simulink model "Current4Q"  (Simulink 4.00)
settings: Solver=ode45  StartTime=0.0  StopTime=0.1  MaxStep=0.000005  RelTol=1e-3
undefined symbols (not defined in the file or in its folder): di, La, Ra, Symmetric, Ts, Ttc, Udc
libraries: simulink3 x1

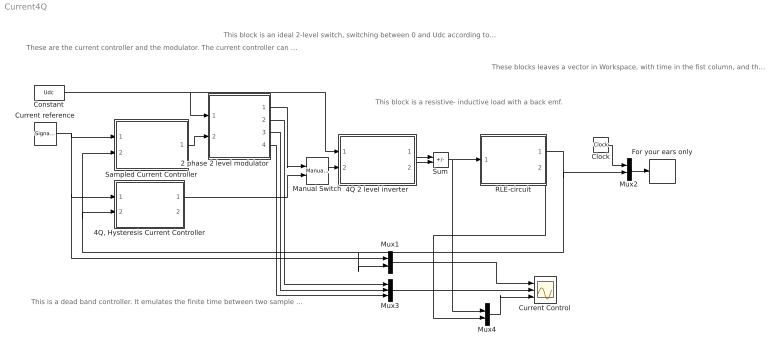
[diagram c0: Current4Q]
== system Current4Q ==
  note: These are the current controller and the modulator. The current controller can emulate several types of controllers.The most didactic is the "fast" but the most realistic is the "slow" and the "slow with Smith Predictor".
  note: This is a dead band controller. It emulates the finite time between two sample time instants, and a dead band.
  note: This block is an ideal 2-level switch, switching between 0 and Udc according to the input signal .
  note: This block is a resistive- inductive load with a back emf.
  note: These blocks leaves a vector in Workspace, with time in the fist column, and the current in the second. Use th file "Playsound" to listen to the sound of the converter, IF you have a sound card in your computer. Type: >>playsound(snd(:,1),snd(:,2))
  2 phase 2 level modulator : Subsystem  mask{Ts=Ts, Random=Fixed frequency, Minswitch=Symmetric}
      mask prompts: Ts "Sampling Interval [s]"; Random "Fixed or random frequency"; Minswitch "Symmetric of Minswitch Modulation"
      mask help: Carrier Wave modulator that uses either fixed frequency modulation or random modulation. The fixed frequency modulation uses 1/(2Ts) as modulation frequency. The random modulation selects the modulatio frequency by random every sampling instant. The selection uses either 1/Ts, 1/(2Ts) or 1/(3Ts) as carrier wave frequency.
      mask init:
      | seed=rand
  4Q 2 level inverter : Subsystem
  "4Q, Hysteresis Current Controller" : Subsystem
  Clock : Clock
  Constant : Constant  Value=Udc
  Current reference : SignalGenerator  WaveForm=square  Amplitude=10  Frequency=20  Units=Hertz
  Current Control : Scope  NumInputPorts=3
  For your ears only : ToWorkspace  VariableName=snd  SampleTime=-1  SaveFormat=Array
  Manual Switch : simulink3/Nonlinear/Manual Switch  sw=1  action=0
  Mux1 : Mux  Inputs=2
  Mux2 : Mux  Inputs=2
  Mux3 : Mux  Inputs=3
  Mux4 : Mux  Inputs=2
  RLE-circuit : Subsystem  mask(RLE-circuit){L=La, R=Ra, e0=40, i0=0}
      mask prompts: L "L [H]"; R "R [ohm]"; e0 "Back emf"; i0 "Starting Current"
      mask help: Parametrar
  Sampled Current Controller : Subsystem  mask{R=Ra, L=La, Kp=(La/Ttc+Ra/2), Ti=La/Ra+Ttc/2, Ttc=Ttc, Umax=Udc, Umin=-Udc, e0=40, SlowFast=Slow Computer with Smith Predictor}
      mask prompts: R "Load resistance"; L "Load inductance"; Kp "Controller gain"; Ti "Integral Time Constant"; Ttc "Sampling time [s]"; Umax "Max output signal"; Umin "Min output signal"; e0 "Starting emf"; SlowFast "Controller type"
  Sum : Sum  Inputs=+-  SaturateOnIntegerOverflow=on
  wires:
  RLE-circuit/1(i) -> Mux2/2, "4Q, Hysteresis Current Controller"/2(i), Sampled Current Controller/2(Act), Mux1/2
  Constant/1 -> 4Q 2 level inverter/1(Udc), 2 phase 2 level modulator/1(udc)
  Clock/1 -> Mux2/1
  Mux2/1 -> For your ears only/1
  Mux1/1 -> Current Control/1
  Mux3/1 -> Current Control/2
  Current reference/1 -> Sampled Current Controller/1(Ref), Mux1/1, "4Q, Hysteresis Current Controller"/1(i*)
  4Q 2 level inverter/1(va) -> Sum/1
  4Q 2 level inverter/2(vb) -> Sum/2
  Sum/1 -> Mux4/1, RLE-circuit/1(u)
  2 phase 2 level modulator/1(sa,b) -> Manual Switch/1
  "4Q, Hysteresis Current Controller"/1(sa,b) -> Manual Switch/2
  Manual Switch/1 -> 4Q 2 level inverter/2(sa,b)
  2 phase 2 level modulator/2(va*) -> Mux3/1
  2 phase 2 level modulator/3(vb*) -> Mux3/2
  2 phase 2 level modulator/4(um) -> Mux3/3
  Sampled Current Controller/1(u*) -> 2 phase 2 level modulator/2(u*)
  Mux4/1 -> Current Control/3
  RLE-circuit/2(" e") -> Mux4/2

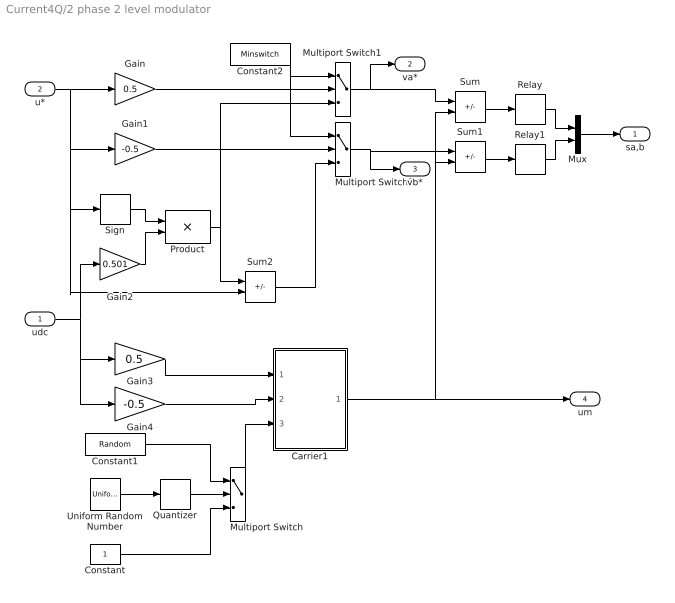
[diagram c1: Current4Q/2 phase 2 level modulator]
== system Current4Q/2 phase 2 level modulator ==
  udc : Inport  Port=1  LatchInput=off
  u* : Inport  Port=2  LatchInput=off
  Carrier1 : Subsystem
  Constant : Constant  Value=1
  Constant1 : Constant  Value=Random
  Constant2 : Constant  Value=Minswitch
  Gain : Gain  Gain=0.5  Multiplication=Element-wise(K.*u)  SaturateOnIntegerOverflow=on
  Gain1 : Gain  Gain=-0.5  Multiplication=Element-wise(K.*u)  SaturateOnIntegerOverflow=on
  Gain2 : Gain  Gain=0.501  Multiplication=Element-wise(K.*u)  SaturateOnIntegerOverflow=on
  Gain3 : Gain  Gain=0.5  Multiplication=Element-wise(K.*u)  SaturateOnIntegerOverflow=on
  Gain4 : Gain  Gain=-0.5  Multiplication=Element-wise(K.*u)  SaturateOnIntegerOverflow=on
  Multiport Switch : MultiPortSwitch  Inputs=2
  Multiport Switch1 : MultiPortSwitch  Inputs=2
  Multiport Switch2 : MultiPortSwitch  Inputs=2
  Mux : Mux  Inputs=2
  Product : Product  Inputs=2  Multiplication=Element-wise(.*)  SaturateOnIntegerOverflow=on
  Quantizer : Quantizer  QuantizationInterval=1  LinearizeAsGain=on
  Relay : Relay  OnSwitchValue=eps  OffSwitchValue=eps  OnOutputValue=1  OffOutputValue=-1
  Relay1 : Relay  OnSwitchValue=eps  OffSwitchValue=eps  OnOutputValue=1  OffOutputValue=-1
  Sign : Signum
  Sum : Sum  Inputs=+-  SaturateOnIntegerOverflow=on
  Sum1 : Sum  Inputs=+-  SaturateOnIntegerOverflow=on
  Sum2 : Sum  Inputs=+-  SaturateOnIntegerOverflow=on
  Uniform Random Number : UniformRandomNumber  Minimum=1  Maximum=3  Seed=seed  SampleTime=Ts
  sa,b : Outport  Port=1  InitialOutput=0
  va* : Outport  Port=2  InitialOutput=0
  vb* : Outport  Port=3  InitialOutput=0
  um : Outport  Port=4  InitialOutput=0
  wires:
  Sum/1 -> Relay/1
  Sum1/1 -> Relay1/1
  u*/1 -> Gain/1, Gain1/1, Sign/1, Sum2/2
  Sign/1 -> Product/1
  udc/1 -> Gain2/1, Gain3/1, Gain4/1
  Gain2/1 -> Product/2
  Product/1 -> Sum2/1, Multiport Switch1/3
  Gain/1 -> Multiport Switch1/2
  Gain1/1 -> Multiport Switch2/2
  Multiport Switch1/1 -> Sum/1, va*/1
  Multiport Switch2/1 -> Sum1/1, vb*/1
  Sum2/1 -> Multiport Switch2/3
  Gain4/1 -> Carrier1/2(Umin)
  Gain3/1 -> Carrier1/1(Umax)
  Quantizer/1 -> Multiport Switch/2
  Uniform Random Number/1 -> Quantizer/1
  Constant/1 -> Multiport Switch/3
  Multiport Switch/1 -> Carrier1/3(x)
  Constant1/1 -> Multiport Switch/1
  Carrier1/1(um) -> Sum1/2, Sum/2, um/1
  Constant2/1 -> Multiport Switch1/1, Multiport Switch2/1
  Relay/1 -> Mux/1
  Relay1/1 -> Mux/2
  Mux/1 -> sa,b/1

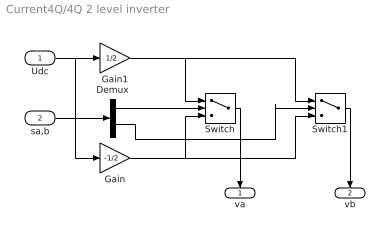
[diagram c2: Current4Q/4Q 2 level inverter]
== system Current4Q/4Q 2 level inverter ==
  Udc : Inport  Port=1  LatchInput=off
  sa,b : Inport  Port=2  LatchInput=off
  Demux : Demux  Outputs=2  BusSelectionMode=off
  Gain : Gain  Gain=-1/2  Multiplication=Element-wise(K.*u)  SaturateOnIntegerOverflow=on
  Gain1 : Gain  Gain=1/2  Multiplication=Element-wise(K.*u)  SaturateOnIntegerOverflow=on
  Switch : Switch  Threshold=0
  Switch1 : Switch  Threshold=0
  va : Outport  Orientation=down  Port=1  InitialOutput=0
  vb : Outport  Orientation=down  Port=2  InitialOutput=0
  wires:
  Gain1/1 -> Switch/1, Switch1/1
  Gain/1 -> Switch/3, Switch1/3
  Switch/1 -> va/1
  Switch1/1 -> vb/1
  Udc/1 -> Gain1/1, Gain/1
  sa,b/1 -> Demux/1
  Demux/1 -> Switch/2
  Demux/2 -> Switch1/2

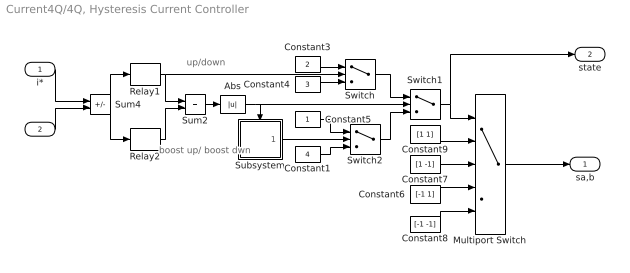
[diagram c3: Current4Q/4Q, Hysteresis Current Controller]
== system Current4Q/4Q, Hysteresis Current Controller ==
  note: up/down
  note: boost up/ boost dwn
  i* : Inport  Port=1  LatchInput=off
  i : Inport  Port=2  LatchInput=off
  Abs : Abs  SaturateOnIntegerOverflow=on
  Constant1 : Constant  Value=4
  Constant3 : Constant  Value=2
  Constant4 : Constant  Value=3
  Constant5 : Constant  Value=1
  Constant6 : Constant  Value=[-1 1]
  Constant7 : Constant  Value=[1 -1]
  Constant8 : Constant  Value=[-1 -1]
  Constant9 : Constant  Value=[1 1]
  Multiport Switch : MultiPortSwitch  Inputs=4
  Relay1 : Relay  OnSwitchValue=di/2  OffSwitchValue=-di/2  OnOutputValue=1  OffOutputValue=-1
  Relay2 : Relay  OnSwitchValue=1.3*di/2  OffSwitchValue=-1.3*di/2  OnOutputValue=1  OffOutputValue=-1
  Subsystem : Subsystem  TreatAsAtomicUnit=on
  Sum2 : Sum  Inputs=++  SaturateOnIntegerOverflow=on
  Sum4 : Sum  Inputs=+-  SaturateOnIntegerOverflow=on
  Switch : Switch  Threshold=0
  Switch1 : Switch  Threshold=1
  Switch2 : Switch  Threshold=0.5
  sa,b : Outport  Port=1
  state : Outport  Port=2
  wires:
  Sum4/1 -> Relay1/1, Relay2/1
  Relay1/1 -> Sum2/1, Switch/2
  Relay2/1 -> Sum2/2
  Sum2/1 -> Abs/1
  Switch/1 -> Switch1/1
  Constant3/1 -> Switch/1
  Constant4/1 -> Switch/3
  Switch1/1 -> Multiport Switch/1, state/1
  Multiport Switch/1 -> sa,b/1
  Abs/1 -> Switch1/2, Subsystem/Trigger
  i*/1 -> Sum4/1
  i/1 -> Sum4/2
  Constant5/1 -> Switch2/1
  Constant1/1 -> Switch2/3
  Switch2/1 -> Switch1/3
  Subsystem/1(Toggle) -> Switch2/2
  Constant6/1 -> Multiport Switch/4
  Constant7/1 -> Multiport Switch/3
  Constant8/1 -> Multiport Switch/5
  Constant9/1 -> Multiport Switch/2

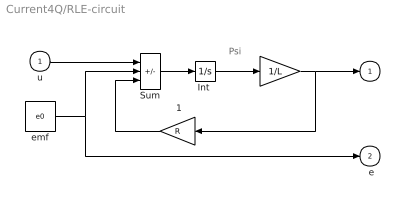
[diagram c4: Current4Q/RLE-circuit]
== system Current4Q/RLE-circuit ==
  note: i
  note: Psi
  u : Inport  Port=1  LatchInput=off
  " " : Gain  Gain=1/L  Multiplication=Element-wise(K.*u)  SaturateOnIntegerOverflow=on
  " 1" : Gain  Orientation=left  Gain=R  Multiplication=Element-wise(K.*u)  SaturateOnIntegerOverflow=on
  "Int " : Integrator  ExternalReset=none  InitialConditionSource=internal  InitialCondition=i0*L  LimitOutput=off  UpperSaturationLimit=inf  LowerSaturationLimit=-inf  ShowSaturationPort=off  ShowStatePort=off  AbsoluteTolerance=auto
  Sum : Sum  Inputs=+--  SaturateOnIntegerOverflow=on
  emf : Constant  Value=e0
  i : Outport  Port=1  InitialOutput=0
  " e" : Outport  Port=2  InitialOutput=0
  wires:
  " "/1 -> i/1, " 1"/1
  " 1"/1 -> Sum/3
  u/1 -> Sum/1
  Sum/1 -> "Int "/1
  "Int "/1 -> " "/1
  emf/1 -> Sum/2, " e"/1

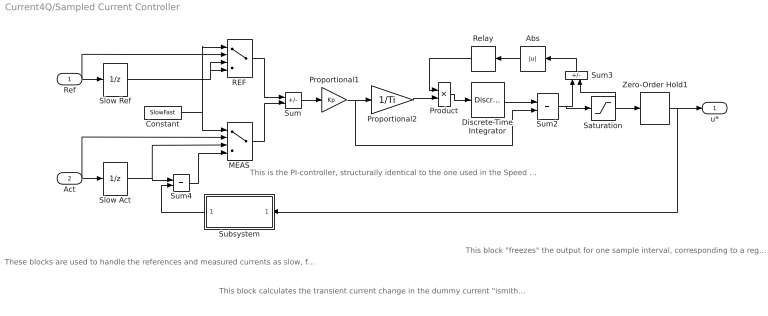
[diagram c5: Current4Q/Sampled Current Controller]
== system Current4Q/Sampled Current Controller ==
  note: These blocks are used to handle the references and measured currents as slow, fast or fast computer with Smith predictor.
  note: This block calculates the transient current change in the dummy current "ismith" The smith predictor calculates the current change that would have been measured if the computer was "fast", i.e. without the delay that a slow computer has. The calculated current change equals the real current change, but informing the controller one sampling interval earlier, thus allowing a high (deadbeat) gain.
  note: This is the PI-controller, structurally identical to the one used in the Speed Controller
  note: This block "freezes" the output for one sample interval, corresponding to a register in a microcontroller where the reference voltages are written once every sampling inteval.
  Ref : Inport  Port=1  LatchInput=off
  Act : Inport  Port=2  LatchInput=off
  Abs : Abs  Orientation=left  SaturateOnIntegerOverflow=on
  Constant : Constant  Value=SlowFast
  Discrete-Time Integrator : DiscreteIntegrator  IntegratorMethod=ForwardEuler  ExternalReset=none  InitialConditionSource=internal  InitialCondition=e0  LimitOutput=on  UpperSaturationLimit=Umax  LowerSaturationLimit=Umin  ShowSaturationPort=off  ShowStatePort=off  SampleTime=Ttc
  MEAS : MultiPortSwitch  Inputs=3
  Product : Product  Inputs=2  Multiplication=Element-wise(.*)  SaturateOnIntegerOverflow=on
  Proportional1 : Gain  Gain=Kp  Multiplication=Element-wise(K.*u)  SaturateOnIntegerOverflow=on
  Proportional2 : Gain  Gain=1/Ti  Multiplication=Element-wise(K.*u)  SaturateOnIntegerOverflow=on
  REF : MultiPortSwitch  Inputs=3
  Relay : Relay  Orientation=left  OnSwitchValue=eps  OffSwitchValue=eps  OnOutputValue=0  OffOutputValue=1
  Saturation : Saturate  UpperLimit=Umax  LowerLimit=Umin  LinearizeAsGain=on
  Slow Act : UnitDelay  X0=0  SampleTime=Ttc
  Slow Ref : UnitDelay  X0=0  SampleTime=Ttc
  Subsystem : Subsystem  Orientation=left
  Sum : Sum  Inputs=+-  SaturateOnIntegerOverflow=on
  Sum2 : Sum  Inputs=++  SaturateOnIntegerOverflow=on
  Sum3 : Sum  Orientation=up  Inputs=+-  SaturateOnIntegerOverflow=on
  Sum4 : Sum  Inputs=++  SaturateOnIntegerOverflow=on
  Zero-Order Hold1 : ZeroOrderHold  SampleTime=Ttc
  u* : Outport  Port=1
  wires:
  Discrete-Time Integrator/1 -> Sum2/1
  Proportional1/1 -> Proportional2/1, Sum2/2
  Sum/1 -> Proportional1/1
  Sum2/1 -> Saturation/1, Sum3/1
  Saturation/1 -> Zero-Order Hold1/1, Sum3/2
  Proportional2/1 -> Product/2
  Product/1 -> Discrete-Time Integrator/1
  Relay/1 -> Product/1
  Ref/1 -> REF/2, Slow Ref/1
  Zero-Order Hold1/1 -> u*/1, Subsystem/1(u)
  Act/1 -> MEAS/2, Slow Act/1
  Slow Act/1 -> Sum4/1, MEAS/3
  Subsystem/1(di_smith) -> Sum4/2
  Constant/1 -> MEAS/1, REF/1
  Slow Ref/1 -> REF/3, REF/4
  REF/1 -> Sum/1
  Sum4/1 -> MEAS/4
  MEAS/1 -> Sum/2
  Sum3/1 -> Abs/1
  Abs/1 -> Relay/1

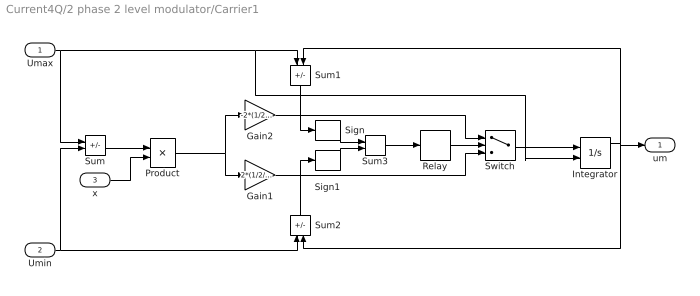
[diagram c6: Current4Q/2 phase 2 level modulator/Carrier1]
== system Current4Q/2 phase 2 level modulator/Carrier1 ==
  Umax : Inport  Port=1  LatchInput=off
  Umin : Inport  Port=2  LatchInput=off
  x : Inport  Port=3  LatchInput=off
  Gain1 : Gain  Gain=2*(1/2/Ts)  Multiplication=Element-wise(K.*u)  SaturateOnIntegerOverflow=on
  Gain2 : Gain  Gain=-2*(1/2/Ts)  Multiplication=Element-wise(K.*u)  SaturateOnIntegerOverflow=on
  Integrator : Integrator  ExternalReset=none  InitialConditionSource=external  InitialCondition=0  LimitOutput=off  UpperSaturationLimit=inf  LowerSaturationLimit=-inf  ShowSaturationPort=off  ShowStatePort=off  AbsoluteTolerance=auto
  Product : Product  Inputs=2  Multiplication=Element-wise(.*)  SaturateOnIntegerOverflow=on
  Relay : Relay  OnSwitchValue=1  OffSwitchValue=-1  OnOutputValue=1  OffOutputValue=-1
  Sign : Signum
  Sign1 : Signum
  Sum : Sum  Inputs=+-  SaturateOnIntegerOverflow=on
  Sum1 : Sum  Orientation=down  Inputs=-+  SaturateOnIntegerOverflow=on
  Sum2 : Sum  Orientation=up  Inputs=-+  SaturateOnIntegerOverflow=on
  Sum3 : Sum  Inputs=++  SaturateOnIntegerOverflow=on
  Switch : Switch  Threshold=0
  um : Outport  Port=1
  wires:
  Switch/1 -> Integrator/1
  Umax/1 -> Sum/1, Sum1/1, Integrator/2
  Umin/1 -> Sum/2, Sum2/1
  Gain2/1 -> Switch/1
  Gain1/1 -> Switch/3
  Integrator/1 -> Sum1/2, um/1, Sum2/2
  Sum1/1 -> Sign/1
  Sum2/1 -> Sign1/1
  Sign/1 -> Sum3/1
  Sign1/1 -> Sum3/2
  Sum3/1 -> Relay/1
  Relay/1 -> Switch/2
  Sum/1 -> Product/1
  Product/1 -> Gain2/1, Gain1/1
  x/1 -> Product/2

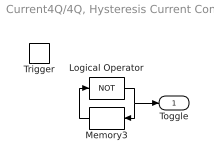
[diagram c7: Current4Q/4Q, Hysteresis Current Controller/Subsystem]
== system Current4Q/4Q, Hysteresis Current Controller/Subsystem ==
  Trigger : TriggerPort  TriggerType=rising  OutputDataType=auto
  Logical Operator : Logic  Operator=NOT  Inputs=2
  Memory3 : Memory  Orientation=left  X0=0  InheritSampleTime=on
  Toggle : Outport  Port=1
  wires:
  Logical Operator/1 -> Memory3/1, Toggle/1
  Memory3/1 -> Logical Operator/1

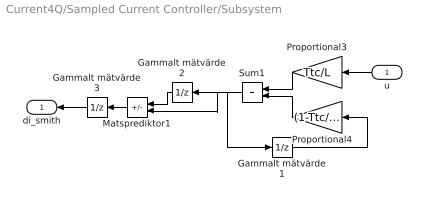
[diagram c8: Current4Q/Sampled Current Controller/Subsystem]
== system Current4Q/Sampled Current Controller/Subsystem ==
  u : Inport  Orientation=left  Port=1  LatchInput=off
  Gammalt mätvärde1 : UnitDelay  X0=e0/R  SampleTime=Ttc
  Gammalt mätvärde2 : UnitDelay  Orientation=left  X0=(1-Ttc/(L/R))*e0/R  SampleTime=Ttc
  Gammalt mätvärde3 : UnitDelay  Orientation=left  X0=e0/R  SampleTime=Ttc
  Matsprediktor1 : Sum  Orientation=left  Inputs=-+  SaturateOnIntegerOverflow=on
  Proportional3 : Gain  Orientation=left  Gain=Ttc/L  Multiplication=Element-wise(K.*u)  SaturateOnIntegerOverflow=on
  Proportional4 : Gain  Orientation=left  Gain=(1-Ttc/(L/R))  Multiplication=Element-wise(K.*u)  SaturateOnIntegerOverflow=on
  Sum1 : Sum  Orientation=left  Inputs=++  SaturateOnIntegerOverflow=on
  di_smith : Outport  Orientation=left  Port=1
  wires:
  Proportional3/1 -> Sum1/1
  Gammalt mätvärde1/1 -> Proportional4/1
  Proportional4/1 -> Sum1/2
  Sum1/1 -> Gammalt mätvärde1/1, Gammalt mätvärde2/1, Matsprediktor1/2
  u/1 -> Proportional3/1
  Gammalt mätvärde2/1 -> Matsprediktor1/1
  Matsprediktor1/1 -> Gammalt mätvärde3/1
  Gammalt mätvärde3/1 -> di_smith/1
